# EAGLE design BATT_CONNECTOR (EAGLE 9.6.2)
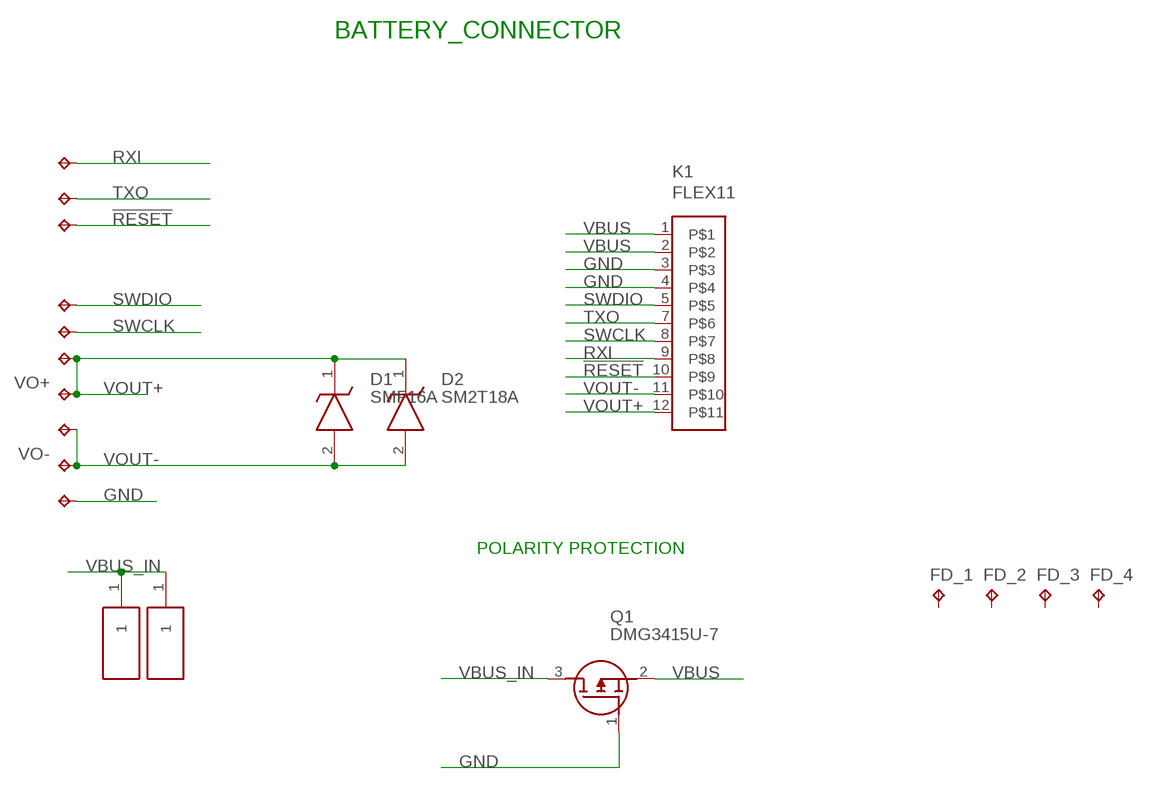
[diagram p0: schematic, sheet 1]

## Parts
!RESET  TPB2,54  [B2,54]
D1  SMF16A  [SODFL3618X110N]
D2  SM2T18A  [SM2T18A]
FD_1  FD_1  TPTP06SQ  [TP06SQ]
FD_2  FD_1  TPTP06SQ  [TP06SQ]
FD_3  FD_1  TPTP06SQ  [TP06SQ]
FD_4  FD_1  TPTP06SQ  [TP06SQ]
GND  TPB2,54  [B2,54]
H1  S1761-42R  [S176142R]
H2  S1761-42R  [S176142R]
K1  FLEX11  [FLEX11]
Q1  DMG3415U-7  SSM3J338R,LF  [SSM3J332RLFT]
RXI  TPB2,54  [B2,54]
SWCLK  TPB2,54  [B2,54]
SWDIO  TPB2,54  [B2,54]
TXO  TPB2,54  [B2,54]
VO+  TPB2,54  [B2,54]
VO-  TPB2,54  [B2,54]
VOUT+1  TPB2,54  [B2,54]
VOUT-1  TPB2,54  [B2,54]

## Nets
!RESET: !RESET.TP K1.10
GND: GND.TP K1.3 K1.4 Q1.1(G)
RXI: K1.9 RXI.TP
SWCLK: K1.8 SWCLK.TP
SWDIO: K1.5 SWDIO.TP
TXO: K1.7 TXO.TP
VBUS: K1.1 K1.2 Q1.2(S)
VBUS_IN: H1.1 H2.1 Q1.3(D)
VOUT+: D1.1(K) D2.1(K) K1.12 VO+.TP VOUT+1.TP
VOUT-: D1.2(A) D2.2(A) K1.11 VO-.TP VOUT-1.TP
Unconnected: FD_1.TP FD_2.TP FD_3.TP FD_4.TP

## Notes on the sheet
- BATTERY_CONNECTOR
- POLARITY PROTECTION

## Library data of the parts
!RESET FD_1-FD_4 GND RXI SWCLK SWDIO TXO VO+ VO- VOUT+1 VOUT-1 = testpad:TP: Test pad
D1 = SMF16A:SMF16A: ESD Suppressors / TVS Diodes 200W 16V 5% Uni-directional; ARROW_PART_NUMBER: SMF16A; ARROW_PRICE-STOCK: https://www.arrow.com/en/products/smf16a/littelfuse; DESCRIPTION: ESD Suppressors / TVS Diodes 200W 16V 5% Uni-directional; HEIGHT: 1.1mm; MANUFACTURER_NAME: LITTELFUSE; MANUFACTURER_PART_NUMBER: SMF16A; MOUSER_PART_NUMBER: 576-SMF16A; MOUSER_PRICE-STOCK: https://www.mouser.co.uk/ProductDetail/Littelfuse/SMF16A?qs=IP%252BaFeBnnar8T%2Ffm%252BJ%2Flrw%3D%3D
D2 = SM2T18A:SM2T18A: 200 W TVS in STmite; DESCRIPTION: 200 W TVS in STmite; HEIGHT: 1.15mm; MANUFACTURER_NAME: STMicroelectronics; MANUFACTURER_PART_NUMBER: SM2T18A; MOUSER_PART_NUMBER: 511-SM2T18A; MOUSER_PRICE-STOCK: https://www.mouser.co.uk/ProductDetail/STMicroelectronics/SM2T18A?qs=9NrABl3fj%2FoQ9e7jVf8sKA%3D%3D
H1 H2 = S1761-42R:S1761-42R: EZ_Boardware SMT Spring Contact 3.5mm; DESCRIPTION: EZ_Boardware SMT Spring Contact 3.5mm; HEIGHT: 3.8mm; MANUFACTURER_NAME: Harwin; MANUFACTURER_PART_NUMBER: S1761-42R; MOUSER_PART_NUMBER: 855-S1761-42R; MOUSER_PRICE-STOCK: https://www.mouser.co.uk/ProductDetail/Harwin/S1761-42R?qs=ulE8k0yEMYZkmoaxRCFkSQ%3D%3D
K1 = Flex_3mm:FLEX11
Q1 = SSM3J338R_LF:SSM3J338R,LF: MOSFET Small-signal MOSFET Vdss= -12V, ID= -6A Source: Datasheet; ARROW_PART_NUMBER: SSM3J338R,LF; ARROW_PRICE-STOCK: https://www.arrow.com/en/products/ssm3j338rlf/toshiba?region=nac; DESCRIPTION: MOSFET Small-signal MOSFET Vdss= -12V, ID= -6A; HEIGHT: mm; MANUFACTURER_NAME: Toshiba; MANUFACTURER_PART_NUMBER: SSM3J338R,LF; MOUSER_PART_NUMBER: 757-SSM3J338RLF; MOUSER_PRICE-STOCK: https://www.mouser.co.uk/ProductDetail/Toshiba/SSM3J338RLF?qs=lhkzy8lC%252BSvURFM9ZjmJSw%3D%3D

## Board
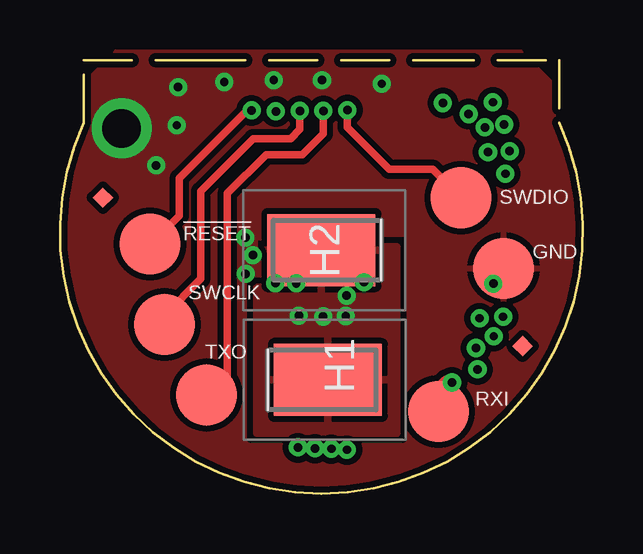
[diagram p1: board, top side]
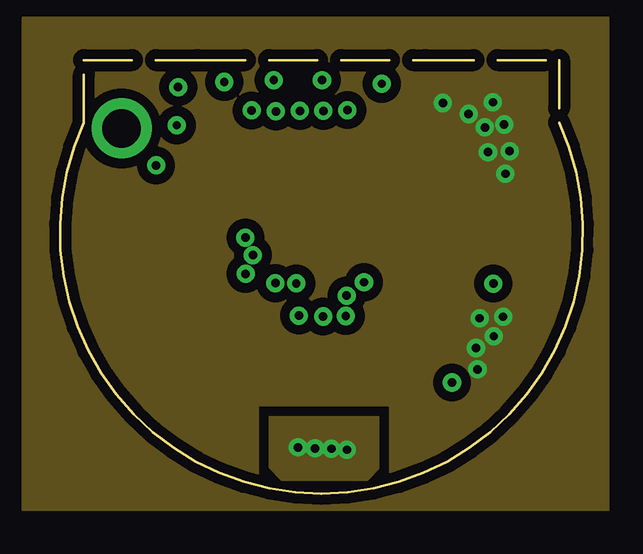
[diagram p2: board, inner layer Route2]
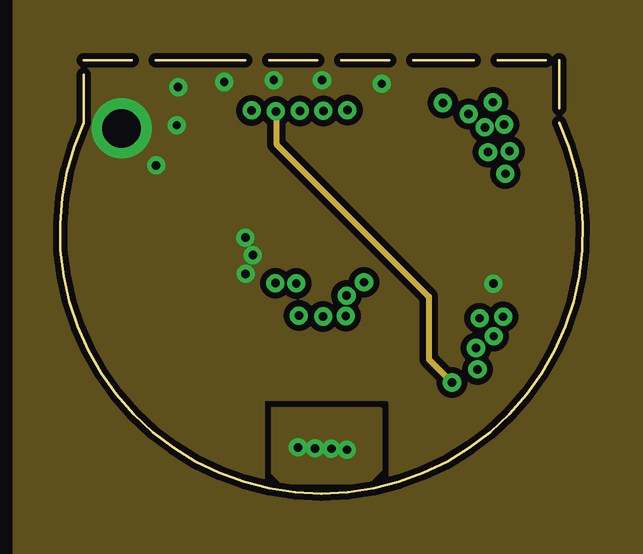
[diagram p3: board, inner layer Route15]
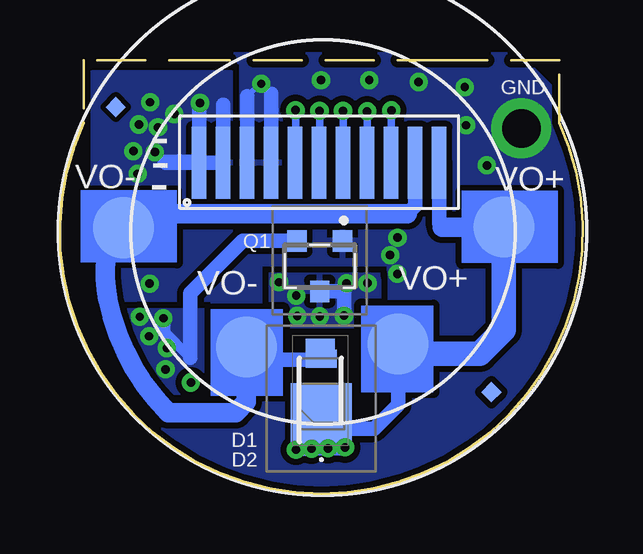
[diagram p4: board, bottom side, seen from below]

Size 21.79 x 18.07 mm. Coordinates in mm from the lower left corner, seen from the top.
Outline: 20.79,18.07 20.79,15.46 arc-229 0.99,15.46 0.99,18.07 5.73,18.07 5.71,18.06 15.21,18.06 15.23,18.07 20.79,18.07
Copper layers (1+2*15+16): Top 0.035mm / dielectric 1.5mm / Route2 0.035mm / dielectric 0.15mm / Route15 0.035mm / dielectric 0.2mm / Bottom 0.035mm
Design rules "default *": minimum track width 0.00038125mm, minimum drill 0.35mm, track to track 8mil, track to pad 8mil, pad to pad 8mil, via to via 8mil, smd to smd 5mil, copper to edge 8mil, drill to drill 8mil, minimum pad ring 10mil, minimum via ring 8mil, stop-mask expansion 2mil, vias tented up to drill 50mil, thermal gap 10mil
bRestrict: area 21,9.5 to 21.7,12.6

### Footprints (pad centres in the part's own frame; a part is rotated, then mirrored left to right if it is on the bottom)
B2,54 = smd 2.54 x 2.54: TP 0,0
SODFL3618X110N = smd 1.2 x 1.22: 1 -1.55,0; 2 1.55,0
SM2T18A = smd 2.67 x 2.54: 1 -0.698,0 | smd 0.762 x 1.27: 2 1.653,0
TP06SQ = smd 0.6 x 0.6: TP 0,0
S176142R = smd 3 x 4.5: 1 0,-2
FLEX11 = smd 0.6 x 3: 1 0.8,2.05; 2 1.8,2.05; 3 2.8,2.05; 4 3.8,2.05; 5 4.8,2.05; 7 5.8,2.05; 8 6.8,2.05; 9 7.8,2.05; 10 8.8,2.05; 11 9.8,2.05; 12 10.8,2.05
SSM3J332RLFT = smd 0.8 x 0.9: 1 -0.95,-1.05; 2 0.95,-1.05; 3 0,1.05

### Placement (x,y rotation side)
!RESET  3.74,10.41 0 top
D1  10.94,4.3 90 bottom
D2  10.89,3.97 90 bottom
FD_1  3.81,4.23 45 bottom
FD_2  19.46,16.11 45 bottom
FD_3  1.78,12.33 45 top
FD_4  19.27,6.15 45 top
GND  18.48,9.39 0 top
H1  13.16,4.74 270 top
H2  8.89,10.15 90 top
K1  16.79,11.73 0 bottom
Q1  10.96,9.48 180 bottom
RXI  15.77,3.42 0 top
SWCLK  4.35,7.05 0 top
SWDIO  16.7,12.33 0 top
TXO  6.1,4.11 0 top
VO+  3.29,11.11 0 bottom
VO-  19.13,11.08 0 bottom
VOUT+1  7.7,6.23 0 bottom
VOUT-1  14.02,6.12 0 bottom

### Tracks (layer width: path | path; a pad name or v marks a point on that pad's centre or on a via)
!RESET  (via drill 0.35)
  Top 0.305: !RESET.TP 3.8,10.41 4.97,11.58 4.97,13.15 7.79,15.97 v7.98,15.97
  Bottom 0.203: K1.10
  Bottom 0.305: v7.98,15.97 K1.10
GND  (via drill 0.35, 1.6 pad 2.5)
  Bottom 0.203: 12.99,16.67 v13.4,17.08 13.47,17.08 13.99,16.56
  Bottom 0.61: 12.99,16.67 K1.4 | 13.99,16.56 K1.3
  other vias: 6.84,17.15 4,13.68 8.03,9.94 7.73,9.16 18.05,8.75 7.72,10.67 4.86,15.35 4.92,16.94 8.9,17.23 10.91,17.23 2.56,15.22
  pour Bottom (isolate 0.254, rank 2): 2.66,18.32 19.36,18.32 22.17,15.51 22.17,-0.48 2.16,-0.48 -1.44,3.12 -1.44,14.22
  pour Top (isolate 0.254, rank 2): 2.29,18.46 19.22,18.46 22.96,14.72 22.96,5.7 16.98,-0.28 3.36,-0.28 -1.32,4.4 -1.32,14.85
  pour Bottom (isolate 0.305): 3.46,17.82 3.46,11.91 6.66,11.91 6.66,17.82
  pour Route15 (isolate 0.254, rank 2): -1.94,20.62 -1.94,-2.48 25.06,-2.48 25.06,20.62
RXI  (via drill 0.35)
  Top 0.61: RXI.TP 15.77,4.28 16.12,4.63 v16.33,4.63
  Route15 0.203: v8.99,15.93 9.01,15.91
  Route15 0.254: v16.33,4.63 15.36,5.6 15.36,8.21 9.01,14.56 9.01,15.91
  Bottom 0.203: v8.99,15.93
  Bottom 0.305: K1.9 v8.99,15.93
SWCLK  (via drill 0.35)
  Top 0.254: SWCLK.TP 4.35,7.44
  Top 0.305: 4.35,7.44 5.86,8.95 5.86,12.6 8.05,14.79 9.6,14.79 9.99,15.18 v9.99,15.95
  Bottom 0.305: v9.99,15.95 K1.8
SWDIO  (via drill 0.35)
  Top 0.305: v11.97,15.98 11.97,15.26 13.72,13.51 15.52,13.51 SWDIO.TP
  Bottom 0.203: 11.97,13.8 K1.5
  Bottom 0.305: v11.97,15.98 11.97,13.8
TXO  (via drill 0.35)
  Top 0.305: TXO.TP 6.23,4.11 6.97,4.85 6.97,12.51 8.58,14.12 10.1,14.12 10.97,15 v10.97,15.95
  Bottom 0.203: 10.97,13.8 K1.7
  Bottom 0.305: v10.97,15.95 10.97,13.8
VBUS  (via drill 0.35)
  Bottom 0.406: 16.35,5.67 17.48,6.8
  Bottom 0.61: Q1.2 14.17,10.53 16.35,8.35 16.35,5.67 | 17.48,6.8 v17.48,7.31 | 14.99,16.21 K1.2 17.38,13.78 17.42,13.82 16.03,13.82 K1.1 15.99,16.24 v15.95,16.28
  other vias: 18.03,16.31 17.02,15.82 17.83,14.23 18.73,14.27 18.5,15.38 18.07,6.56 18.46,7.37 17.33,6.07 17.39,5.18 18.55,13.33 17.7,15.26
  pour Route2 (isolate 0.406, rank 2): -1.57,19.82 -1.57,-0.68 22.87,-0.68 22.87,19.82
  pour Bottom: 14.63,17.62 14.63,12.13 20.46,12.13 20.46,17.62
  pour Bottom (isolate 0.254): 15.38,7.71 15.38,4.15 19.16,4.15 19.16,7.71
VBUS_IN  (via drill 0.35)
  Bottom 0.61: Q1.3 10.06,8.43 9.95,8.32 v9.95,7.42
  other vias: 10.96,7.38 9.84,8.76 11.9,7.4 11.94,8.25 8.97,8.77 12.66,8.81
  pour Top: 8.2,10.29 14.02,10.29 14.02,2.51 8.2,2.51
  pour Bottom (isolate 0.305): 8.42,9.17 13.07,9.17 13.07,6.93 8.42,6.93
VOUT+  (via drill 0.35)
  Bottom 0.152: D2.1 10.94,3.22 D1.1
  Bottom 0.61: VOUT+1.TP 7.7,3.7 8.7,2.71 10.94,2.71 D1.1 9.76,2.75 v10.62,1.89 | 5.85,11.11 5.99,11.25 K1.12 | v10.62,1.89 9.95,1.89 v9.91,1.93 | v10.62,1.89 11.28,1.89 v11.3,1.87 11.91,1.87 v11.95,1.83
  Bottom 0.813: VO+.TP 5.85,11.11
  Bottom 1.016: VOUT+1.TP 7.3,5.83 4.3,5.83 3.29,6.84 VO+.TP
  pour Route2 (isolate 0.254): 8.71,1.1 9.22,0.59 12.81,0.59 13.27,1.05 13.27,3.19 8.71,3.19
  pour Route15 (isolate 0.254): 8.82,3.58 8.82,0.85 9.21,0.46 9.24,0.43 12.57,0.43 12.83,0.43 13.4,1 13.4,3.52 13.37,3.55 8.85,3.55
VOUT-
  Bottom 0.152: VO-.TP 19.17,11.12 19.56,11.12 | D2.2 10.89,5.8 D1.2
  Bottom 0.406: VOUT-1.TP 14.02,5.57 | D1.2 11.24,5.57
  Bottom 0.61: 14.02,5.57 11.24,5.57 | K1.11 6.99,11.99 7.32,11.66
  Bottom 0.813: VOUT-1.TP 14.02,3.83 14.47,3.38 17.27,3.38 arc34 19.8,8.09 arc32 19.56,11.12 | VO-.TP 18.55,11.66 7.32,11.66
  Bottom 1.016: 19.13,10.46 VO-.TP
(copper drawn outside any net)
  shapes: Bottom area x4

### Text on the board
bNames: GND | - | - | - | VO+ | VO-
